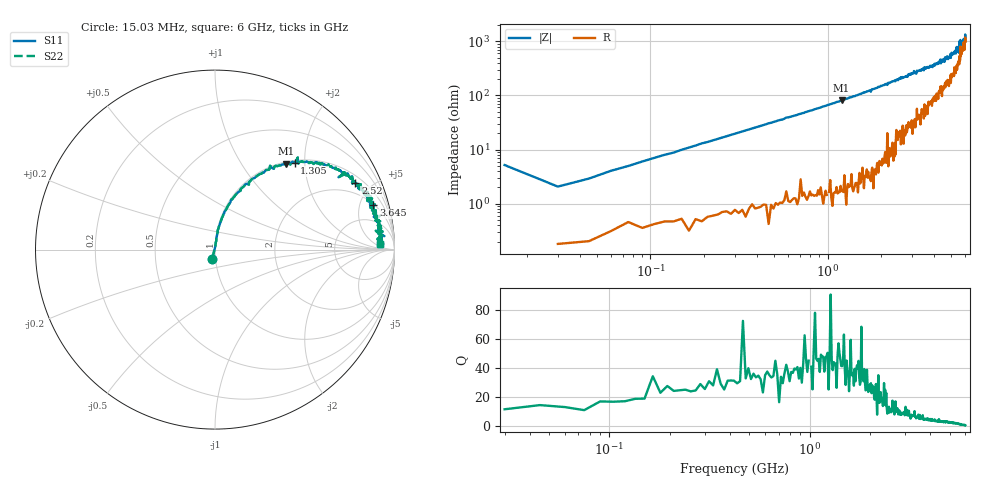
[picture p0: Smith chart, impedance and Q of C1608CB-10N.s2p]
!	Network	Analyzer	HP8753E.07.74:	Oct	30	2002	Serial	No.	JP38451487
!	Hewlett-Packard
!	7	Sep	2009	9:34:10
!	Frequency	S11	S21	S12	S22
#	HZ	S	RI	R	50
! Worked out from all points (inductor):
!   400 points, 15.03 MHz to 6 GHz, reference 50 ohm
!   read as one part in series: L = 10.5 nH near 45.03 MHz
!   highest Q = 47.8 at 1.2 GHz (marker M1), where L = 10.7 nH
!   S11 on the Smith chart (normalised r, x): 15.03 MHz: 0.97, -0.10; 1.305 GHz: 1.05, +1.78; 2.52 GHz: 1.35, +4.01; 3.645 GHz: 2.11, +6.60; 6 GHz: 21, +8
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1.502992e7  -0.0151 -0.0499  1.02 0.0499  1.02 0.0499  -0.0151 -0.0499
3.002985e7  0.00247 0.0206  0.998 -0.0206  0.998 -0.0206  0.00247 0.0206
6.00297e7  0.00453 0.0403  0.995 -0.0403  0.995 -0.0403  0.00453 0.0403
1.200294e8  0.0109 0.0787  0.989 -0.0787  0.989 -0.0787  0.0109 0.0787
2.850286e8  0.0397 0.179  0.96 -0.179  0.96 -0.179  0.0397 0.179
5.850271e8  0.143 0.329  0.857 -0.329  0.857 -0.329  0.143 0.329
1.020025e9  0.319 0.454  0.681 -0.454  0.681 -0.454  0.319 0.454
1.200024e9  0.398 0.479  0.602 -0.479  0.602 -0.479  0.398 0.479
1.305023e9  0.444 0.484  0.556 -0.484  0.556 -0.484  0.444 0.484
2.01002e9  0.685 0.446  0.315 -0.446  0.315 -0.446  0.685 0.446
2.520017e9  0.782 0.371  0.218 -0.371  0.218 -0.371  0.782 0.371
3.015015e9  0.851 0.32  0.149 -0.32  0.149 -0.32  0.851 0.32
3.645012e9  0.883 0.248  0.117 -0.248  0.117 -0.248  0.883 0.248
4.00501e9  0.896 0.217  0.104 -0.217  0.104 -0.217  0.896 0.217
5.010005e9  0.914 0.141  0.0862 -0.141  0.0862 -0.141  0.914 0.141
5.355003e9  0.934 0.0999  0.0656 -0.0999  0.0656 -0.0999  0.934 0.0999
5.535002e9  0.896 0.105  0.104 -0.105  0.104 -0.105  0.896 0.105
5.565002e9  0.944 0.0748  0.0561 -0.0748  0.0561 -0.0748  0.944 0.0748
5.595002e9  0.908 0.0924  0.092 -0.0924  0.092 -0.0924  0.908 0.0924
5.625002e9  0.93 0.0538  0.0696 -0.0538  0.0696 -0.0538  0.93 0.0538
5.655002e9  0.92 0.0793  0.0803 -0.0793  0.0803 -0.0793  0.92 0.0793
6e9  0.919 0.0298  0.0807 -0.0298  0.0807 -0.0298  0.919 0.0298
